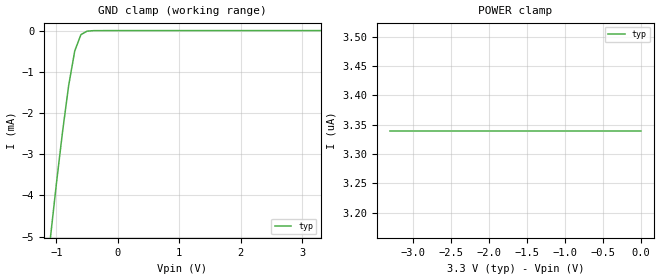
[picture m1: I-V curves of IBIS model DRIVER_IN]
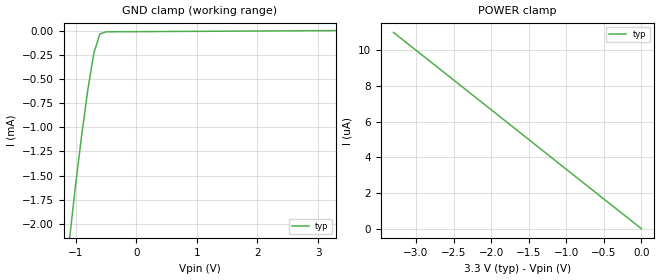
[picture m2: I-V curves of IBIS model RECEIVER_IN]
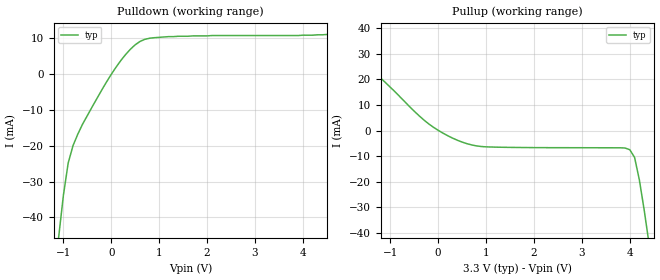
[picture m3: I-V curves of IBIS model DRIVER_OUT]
|   Texas Instruments Incorporated
|   Data Transmissions Products
|   IBIS Model for SN65LVM179
|   8D SOIC Package
[IBIS Ver]   2.1
[Comment char]   |_char
[File name]   lvdm179.ibs
[File Rev]   2.0
[Date]   5Jan99
[Source]   File originated at Texas Instruments Incorporated.
   Data Transmission Products Group.
[Notes]
[Disclaimer]
(C) Copyright Texas Instruments Incorporated 1999
   All rights reserved
  Texas Instruments Incorporated hereby grants the user of this IBIS
model a non-exclusive, nontransferable license to use this IBIS model
under the following terms.  Before using this IBIS model, the user
should read this license.  If the user does not accept these terms,
the IBIS model should be returned to Texas Instruments within 30 days.
  The user is granted this license only to use the IBIS model and
is not granted rights to sell, load, rent, lease or license the IBIS
model in whole or in part, or in modified form to anyone other than
user.  User may modify the IBIS model to suit its specific applications
but rights to derivative works and such modifications shall belong to
Texas Instruments.
  This IBIS model is provided on an "AS IS" basis and Texas Instruments
makes absolutely no warranty with respect to the information contained
herein.  TEXAS INSTRUMENTS DISCLAIMS AND CUSTOMER WAIVES ALL WARRANTIES,
EXPRESS OR IMPLIED, INCLUDING WARRANTIES OF MERCHANTABILITY OR FITNESS
FOR A PARTICULAR PURPOSE. The entire risk as to quality and performance
is with the Customer. ACCORDINGLY, IN NO EVENT SHALL THE COMPANY BE LIABLE
FOR ANY DAMAGES, WHETHER IN CONTRACT OR TORT,INCLUDING ANY LOST PROFITS
OR OTHER INCIDENTAL, CONSEQUENTIAL, EXEMPLARY, OR PUNITIVE DAMAGES ARISING
OUT OF THE USE OR APPLICATION OF THE IBIS model provided in this package.
Further, Texas Instruments reserves the right to discontinue or make changes
without notice to any product herein to improve reliability, function, or
design. Texas Instruments does not convey any license under patent rights
or any other intellectual property rights, including those of third parties.
Contact Texas Instruments at ATTN:DATA TRANSMISSIONS
Thomas Fisher 8505 Forest Lane, M/S 8710, Dallas, TX 75243-4136
[Copyright]   Copyright 1999, Texas Instruments, All Rights Reserved
[Component]   LVDM179D
[Manufacturer]  Texas Instruments Incorporated
[Package]
|   typ   min   max
R_pkg   0.036   0.033   0.039
L_pkg   3.340nH   2.445nH   4.233nH
C_pkg   0.470pF   0.308pF   0.631pF
[Pin]   signal_name   model_name   R_pin   L_pin   C_pin
1   VCC   POWER   0.034   4.233n   0.630p
2   R   RECEIVER_OUT   0.038   2.445n   0.309p
3   D   DRIVER_IN   0.039   2.448n   0.309p
4   GND   GND   0.033   4.231n   0.631p
5   Y   DRIVER_OUT   0.033   4.230n   0.630p
6   Z   DRIVER_OUT   0.039   2.450n   0.308p
7   B   RECEIVER_IN   0.039   2.448n   0.309p
8   A   RECEIVER_IN   0.033   4.231n   0.630p
[Diff_pin]   inv_pin   vdiff   tdelay_typ   tdelay_min   tdelay_max
| The 'A' pin is Diff_pin and the 'B' pin is the inv_pin
8   7   0.100   0 0 0
| Models and submodels in the file (4): DRIVER_IN (Input), RECEIVER_IN (Input), DRIVER_OUT (Output), RECEIVER_OUT (Output)
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|   Driver Input MODEL
[Model]   DRIVER_IN
Model_type   Input
|Signals   D
Vinh = 2.0
Vinl = 0.8
|   typ   min   max
C_comp   1.0pF   NA   NA
|   typ   min   max
[Temperature Range]   25.0   NA   NA
[Voltage range]   3.3V   3.0V   3.6V
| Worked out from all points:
|   GND clamp passes 1 mA (typ) near -0.76 V on its own axis
[GND_clamp]
|   Voltage   I(typ)   I(min)   I(max)
-3.3V     -43.1mA    NA         NA
-1.1V     -5.08mA    NA         NA
-1V       -3.73mA    NA         NA
-900mV    -2.47mA    NA         NA
-800mV    -1.34mA    NA         NA
-700mV    -493uA     NA         NA
-600mV    -98.5uA    NA         NA
-500mV    -13.3uA    NA         NA
3.3V      3.34pA     NA         NA
[Power_clamp]
| Note that the[POWER_clamp]voltage table is referenced to Vcc
| and is calculated using Vtable=Vcc - Vmeasured.
|   Voltage   I(typ)   I(min)   I(max)
-3.3V     3.34uA     NA         NA
-2.7V     3.34uA     NA         NA
-2V       3.34uA     NA         NA
-800mV    3.34uA     NA         NA
0V        3.34uA     NA         NA
|   Receiver Input MODEL
[Model]   RECEIVER_IN
Model_type   Input
|Signals   A,B
Vinh = 2.0
Vinl = 0.8
|   typ   min   max
C_comp   1.0pF   NA   NA
|   typ   min   max
[Temperature Range]   25.0   NA   NA
[Voltage range]   3.3V   3.0V   3.6V
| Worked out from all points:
|   GND clamp passes 1 mA (typ) near -0.88 V on its own axis
[GND_clamp]
|   Voltage   I(typ)   I(min)   I(max)
-3.3V     -22.5mA    NA         NA
-1.1V     -2.15mA    NA         NA
-1V       -1.59mA    NA         NA
-900mV    -1.08mA    NA         NA
-800mV    -616uA     NA         NA
-700mV    -234uA     NA         NA
-600mV    -34.5uA    NA         NA
-500mV    -13.2uA    NA         NA
-400mV    -12.3uA    NA         NA
3.3V      444pA      NA         NA
[Power_clamp]
| Note that the[POWER_clamp]voltage table is referenced to Vcc
| and is calculated using Vtable=Vcc - Vmeasured.
|   Voltage   I(typ)   I(min)   I(max)
-3.3V     11uA       NA         NA
-2V       6.67uA     NA         NA
-1V       3.33uA     NA         NA
0V        0A         NA         NA
|   Driver Output  MODEL
[Model]   DRIVER_OUT
Model_type   Output
| Signals   Y,Z
Vmeas = 1.2V   |Reference voltage for timing measurements
Cref = 5pF   |Timing specification test load capacitance value
Rref = 50   |Note: 50 Ohm load; single ended configuration
Vref = 1.18V   |Timing specification test load voltage
| variable   typ   min   max
C_comp   1.0pF   NA   NA
|   typ   min   max
[Temperature Range]   25.0   NA   NA
[Voltage range]   3.3V   3.0V   3.6V
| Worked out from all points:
|   slope of the pulldown table from 0 to 0.495 V, typ, clamps not added: 60.6 ohm
|   slope of the pullup table from 0 to 0.495 V, typ, clamps not added: 109 ohm
[Pulldown]
|   Voltage   I(typ)   I(min)   I(max)
-3.3V     -370mA     NA         NA
-1.1V     -45.6mA    NA         NA
-1V       -33.8mA    NA         NA
-900mV    -24.8mA    NA         NA
-800mV    -20mA      NA         NA
-700mV    -16.8mA    NA         NA
-300mV    -6.83mA    NA         NA
100mV     1.91mA     NA         NA
400mV     6.9mA      NA         NA
700mV     9.65mA     NA         NA
1.4V      10.5mA     NA         NA
6.6V      12.4mA     NA         NA
[Pullup]
|   Voltage   I(typ)   I(min)   I(max)
| Note that the[Pullup]voltage table is referenced to Vcc
| and is calculated using Vtable=Vcc - Vmeasured.
-3.3V     64.5mA     NA         NA
-2.2V     40.1mA     NA         NA
-400mV    5.79mA     NA         NA
0V        84.2uA     NA         NA
500mV     -4.51mA    NA         NA
1V        -6.37mA    NA         NA
4V        -7.49mA    NA         NA
4.1V      -10.5mA    NA         NA
4.2V      -19.3mA    NA         NA
4.3V      -31mA      NA         NA
4.4V      -43.9mA    NA         NA
6.6V      -370mA     NA         NA
[Ramp]
|   typ   min   max
dV/dt_r   0.314/1ps   NA   NA
dV/dt_f   0.443/1ps   NA   NA
R_load = 50ohm | Note: The measurement is on a differential configuration
